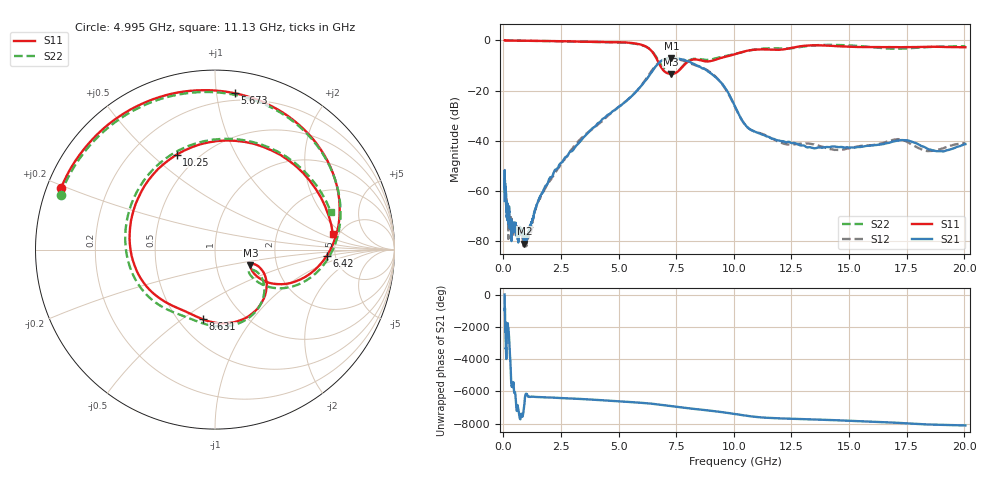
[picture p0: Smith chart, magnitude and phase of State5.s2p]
# Hz S DB R 50
!freq MagS11 AngS11 MagS21 AngS21 MagS12 AngS12 MagS22 AngS22
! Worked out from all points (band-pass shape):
!   1601 points, 50 MHz to 20.05 GHz, reference 50 ohm
!   highest |S21| = -6.93 dB at 7.292 GHz (marker M1); lowest = -81.0 dB at 908.3 MHz (marker M2)
!   |S21| within 3 dB of the highest: 6.646 GHz to 8.375 GHz (1.728 GHz wide, 23 % of centre)
!   lowest |S11| = -13.3 dB at 7.265 GHz (marker M3), VSWR 1.55, Z = 73.2 - j13.3 ohm
!   |S11| at or under -10 dB: 6.802 GHz to 7.82 GHz (1.018 GHz wide, 13.9 % of centre)
!   |S22| runs from -13.0 to 0.0 dB; largest |S21 - S12| = 0.026
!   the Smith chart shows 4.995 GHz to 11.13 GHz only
!   S11 on the Smith chart (normalised r, x): 4.995 GHz: 0.04, +0.19; 5.673 GHz: 0.15, +1.13; 6.42 GHz: 4.26, -0.48; 8.631 GHz: 0.65, -0.60; 10.25 GHz: 0.38, +0.60; 11.13 GHz: 4.49, +1.37
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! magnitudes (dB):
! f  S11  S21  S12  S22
! 50 MHz  0.0  -64.0  -59.4  0.0
! 55.74 MHz  0.0  -52.0  -57.8  0.0
! 135.9 MHz  0.0  -68.1  -66.6  0.0
! 195.5 MHz  0.0  -70.3  -70.3  0.0
! 209.2 MHz  0.0  -72.3  -78.3  0.0
! 251.3 MHz  0.0  -67.9  -70.7  0.0
! 341.7 MHz  0.0  -78.4  -71.2  0.0
! 369.6 MHz  0.0  -72.6  -74.9  0.0
! 908.3 MHz  -0.1  -81.0  -79.9  -0.1
! 1.005 GHz  -0.1  -77.9  -81.0  -0.1
! 2.722 GHz  -0.3  -46.5  -46.4  -0.4
! 4.995 GHz  -0.7  -26.6  -26.5  -0.8
! 5.673 GHz  -1.1  -21.2  -21.2  -1.2
! 6.42 GHz  -4.1  -12.8  -12.2  -4.0
! 7.265 GHz  -13.3  -6.9  -7.1  -12.9
! 7.292 GHz  -13.3  -6.9  -7.1  -12.9
! 7.402 GHz  -13.2  -6.9  -7.2  -13.0
! 8.631 GHz  -8.1  -11.1  -10.9  -7.6
! 10.25 GHz  -4.9  -30.1  -30.2  -4.9
! 11.13 GHz  -3.6  -37.1  -36.9  -3.4
! 14.42 GHz  -2.2  -42.4  -43.6  -1.8
! 20.05 GHz  -2.7  -41.3  -40.9  -2.3
